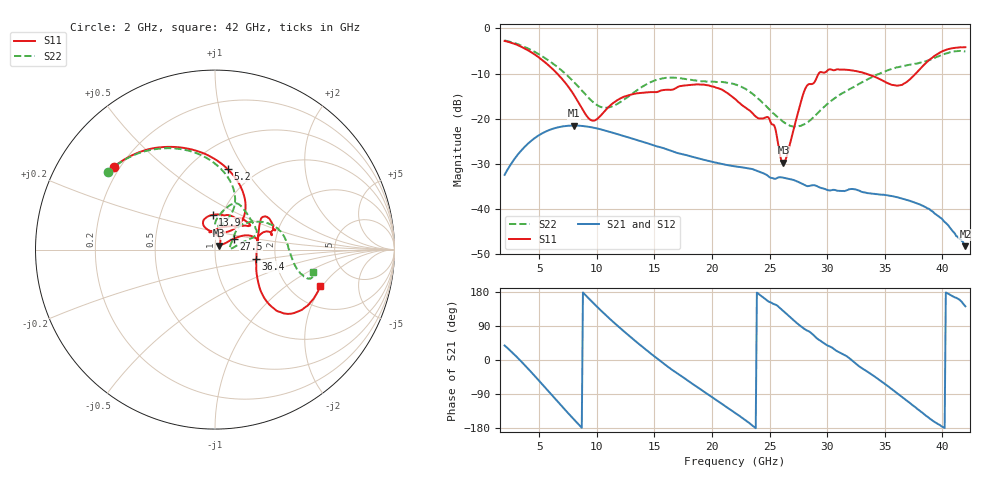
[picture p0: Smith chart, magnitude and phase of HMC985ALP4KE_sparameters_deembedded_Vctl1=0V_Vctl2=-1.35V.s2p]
!s2p File: Measurements: S11, S21, S12, S22
# GHz S dB R 50.0
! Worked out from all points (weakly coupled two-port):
!   401 points, 2 GHz to 42 GHz, reference 50 ohm
!   highest |S21| = -21.53 dB at 8 GHz (marker M1); lowest = -48.3 dB at 42 GHz (marker M2)
!   lowest |S11| = -29.8 dB at 26.2 GHz (marker M3), VSWR 1.07, Z = 52.4 + j2.3 ohm
!   |S11| at or under -10 dB: 6.563 GHz to 29.27 GHz (22.71 GHz wide, 127 % of centre); 33.35 GHz to 37.69 GHz (4.34 GHz wide, 12.2 % of centre)
!   |S22| runs from -21.8 to -2.7 dB; largest |S21 - S12| = 0.00013
!   S11 on the Smith chart (normalised r, x): 2 GHz: 0.18, +0.35; 5.2 GHz: 0.75, +0.84; 13.9 GHz: 0.90, +0.36; 27.5 GHz: 1.22, +0.15; 36.4 GHz: 1.58, -0.18; 42 GHz: 2.91, -1.91
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2  -2.75 140.7  -32.47 38.3  -32.47 38.3  -2.65 143.9
3.5  -4.13 113.0  -26.91 -5.7  -26.92 -5.7  -3.84 119.0
5.2  -6.86 81.0  -23.34 -61.9  -23.35 -61.9  -6.06 92.9
8  -14.65 46.0  -21.53 -156.2  -21.54 -156.3  -11.81 65.7
8.7  -17.68 51.9  -21.61 -178.7  -21.61 -178.7  -13.74 65.9
9.7  -20.46 84.9  -21.99 150.3  -21.99 150.3  -16.38 73.4
10.8  -18.00 112.4  -22.69 118.0  -22.69 118.0  -17.58 86.0
13.9  -14.26 93.9  -25.07 36.3  -25.07 36.3  -13.00 77.7
15.4  -13.94 73.0  -26.26 0.4  -26.26 0.4  -11.24 68.5
19.4  -12.52 34.5  -29.18 -85.5  -29.19 -85.5  -11.73 37.2
22  -15.63 52.3  -30.56 -139.2  -30.57 -139.1  -12.39 19.4
25  -20.16 98.0  -33.00 153.0  -33.01 153.0  -18.00 10.9
26.2  -29.78 42.4  -33.09 128.6  -33.10 128.6  -20.72 3.8
27.5  -18.39 29.9  -34.04 94.3  -34.03 94.1  -21.71 6.7
28.1  -13.35 20.8  -34.78 80.3  -34.80 80.2  -21.13 14.6
28.7  -12.30 12.9  -34.78 69.1  -34.78 69.1  -19.95 23.4
31  -9.08 23.4  -36.01 21.3  -36.02 21.3  -14.86 43.7
33.3  -9.95 34.4  -36.38 -26.9  -36.43 -27.2  -11.59 35.9
35.4  -12.27 12.3  -37.09 -72.1  -37.08 -72.1  -9.17 22.9
36.4  -12.57 -12.9  -37.66 -95.4  -37.68 -95.5  -8.40 15.4
39.5  -5.80 -43.3  -41.34 -166.5  -41.31 -167.3  -6.31 -14.3
42  -4.14 -19.0  -48.29 141.6  -48.45 140.7  -5.06 -12.7
